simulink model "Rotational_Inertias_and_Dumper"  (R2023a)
settings: Solver=VariableStepAuto  StartTime=0.0  StopTime=10.0  RelTol=1e-3
libraries: fl_lib x10, nesl_utility x2

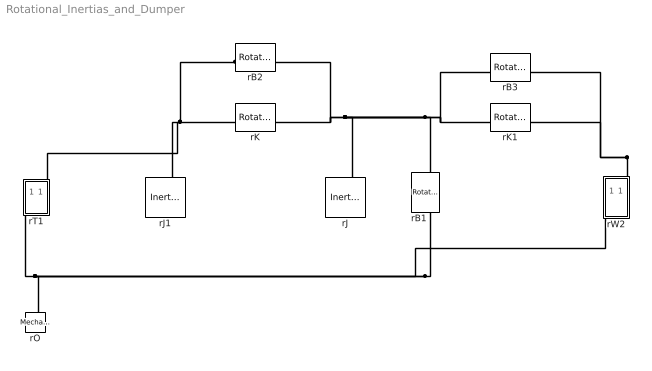
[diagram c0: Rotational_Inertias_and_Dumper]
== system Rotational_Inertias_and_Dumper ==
  rB1 : fl_lib/Mechanical/Rotational Elements/Rotational Damper  D=0.001 N*m*s/rad  w_specify=off  w_priority=None  w=0 rad/s  w_nominal_specify=off  w_nominal_unit=rad/s  w_nominal_value=1  t_specify=off  t_priority=None  t=0 N*m  t_nominal_specify=off  t_nominal_unit=N*m  t_nominal_value=1
  rB2 : fl_lib/Mechanical/Rotational Elements/Rotational Damper  D=0.001 N*m*s/rad  w_specify=off  w_priority=None  w=0 rad/s  w_nominal_specify=off  w_nominal_unit=rad/s  w_nominal_value=1  t_specify=off  t_priority=None  t=0 N*m  t_nominal_specify=off  t_nominal_unit=N*m  t_nominal_value=1
  rB3 : fl_lib/Mechanical/Rotational Elements/Rotational Damper  D=0.001 N*m*s/rad  w_specify=off  w_priority=None  w=0 rad/s  w_nominal_specify=off  w_nominal_unit=rad/s  w_nominal_value=1  t_specify=off  t_priority=None  t=0 N*m  t_nominal_specify=off  t_nominal_unit=N*m  t_nominal_value=1
  rJ : fl_lib/Mechanical/Rotational Elements/Inertia  inertia=0.01 kg*m^2  num_ports=foundation.enum.numPorts2.one  w_specify=off  w_priority=High  w=0 rad/s  w_nominal_specify=off  w_nominal_unit=rad/s  w_nominal_value=1  t_specify=off  t_priority=None  t=0 N*m  t_nominal_specify=off  t_nominal_unit=N*m  t_nominal_value=1
  rJ1 : fl_lib/Mechanical/Rotational Elements/Inertia  inertia=0.01 kg*m^2  num_ports=foundation.enum.numPorts2.one  w_specify=off  w_priority=High  w=0 rad/s  w_nominal_specify=off  w_nominal_unit=rad/s  w_nominal_value=1  t_specify=off  t_priority=None  t=0 N*m  t_nominal_specify=off  t_nominal_unit=N*m  t_nominal_value=1
  rK : fl_lib/Mechanical/Rotational Elements/Rotational Spring  spr_rate=10 N*m/rad  w_specify=off  w_priority=None  w=0 rad/s  w_nominal_specify=off  w_nominal_unit=rad/s  w_nominal_value=1  t_specify=off  t_priority=None  t=0 N*m  t_nominal_specify=off  t_nominal_unit=N*m  t_nominal_value=1  phi_specify=off  phi_priority=High  phi=0 rad  phi_nominal_specify=off  phi_nominal_unit=rad  phi_nominal_value=1
  rK1 : fl_lib/Mechanical/Rotational Elements/Rotational Spring  spr_rate=10 N*m/rad  w_specify=off  w_priority=None  w=0 rad/s  w_nominal_specify=off  w_nominal_unit=rad/s  w_nominal_value=1  t_specify=off  t_priority=None  t=0 N*m  t_nominal_specify=off  t_nominal_unit=N*m  t_nominal_value=1  phi_specify=off  phi_priority=High  phi=0 rad  phi_nominal_specify=off  phi_nominal_unit=rad  phi_nominal_value=1
  rO : fl_lib/Mechanical/Rotational Elements/Mechanical Rotational Reference
  rT1 : Subsystem  mask{rT='Ta'}
      mask prompts: rT "Output variable"
  rW2 : Subsystem  mask{rW='Wa'}
      mask prompts: rW "Output variable"
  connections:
  rB1/RConn1 -- rW2/RConn1 -- rO/LConn1 -- rT1/RConn1
  rB2/LConn1 -- rK/LConn1 -- rJ1/LConn1 -- rT1/LConn1
  rB3/LConn1 -- rB1/LConn1 -- rK1/LConn1 -- rB2/RConn1 -- rK/RConn1 -- rJ/LConn1
  rW2/LConn1 -- rB3/RConn1 -- rK1/RConn1

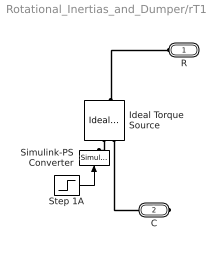
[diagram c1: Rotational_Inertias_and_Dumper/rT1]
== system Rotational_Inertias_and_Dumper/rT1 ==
  Ideal Torque Source : fl_lib/Mechanical/Mechanical Sources/Ideal Torque Source
  Simulink-PS Converter : nesl_utility/Simulink-PS Converter  PhysicalDomain=network_engine_domain  SubClassName=ps_input  LeftPortType=input  RightPortType=output  PseudoPeriodic=off  Frequencies=[]  NoiseDistribution=none  NoiseParameters=[]  Unit=1  AffineConversion=off  FilteringAndDerivatives=zero  SimscapeFilterOrder=1  InputFilterTimeConstant=.001  UdotUserProvided=0
  Step 1A : Step  After=100  SampleTime=0
  R : PMIOPort  Side=Left
  C : PMIOPort  Port=2  Side=Right
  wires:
  Step 1A/1 -> Simulink-PS Converter/1
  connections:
  Ideal Torque Source/RConn2 -- C/RConn1
  Ideal Torque Source/LConn1 -- R/RConn1
  Ideal Torque Source/RConn1 -- Simulink-PS Converter/RConn1

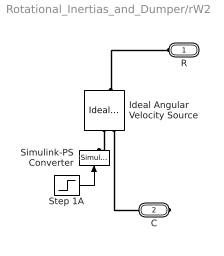
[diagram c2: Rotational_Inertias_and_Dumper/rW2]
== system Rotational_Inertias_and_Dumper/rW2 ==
  Ideal Angular Velocity Source : fl_lib/Mechanical/Mechanical Sources/Ideal Angular Velocity Source
  Simulink-PS Converter : nesl_utility/Simulink-PS Converter  PhysicalDomain=network_engine_domain  SubClassName=ps_input  LeftPortType=input  RightPortType=output  PseudoPeriodic=off  Frequencies=[]  NoiseDistribution=none  NoiseParameters=[]  Unit=1  AffineConversion=off  FilteringAndDerivatives=zero  SimscapeFilterOrder=1  InputFilterTimeConstant=.001  UdotUserProvided=0
  Step 1A : Step  After=100  SampleTime=0
  R : PMIOPort  Side=Left
  C : PMIOPort  Port=2  Side=Right
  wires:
  Step 1A/1 -> Simulink-PS Converter/1
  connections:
  Ideal Angular Velocity Source/RConn2 -- C/RConn1
  Ideal Angular Velocity Source/LConn1 -- R/RConn1
  Ideal Angular Velocity Source/RConn1 -- Simulink-PS Converter/RConn1
